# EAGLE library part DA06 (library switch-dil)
DIL/CODE SWITCH
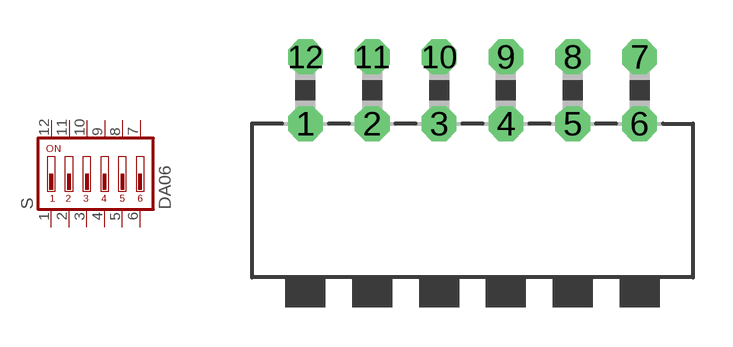
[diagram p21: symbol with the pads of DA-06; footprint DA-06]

Designator prefix S

## DA06 (MPN: MCDA06; OC_FARNELL: 9471553; OC_NEWARK: 26M1091)  [DA-06]
1  1  pas
2  2  pas
3  3  pas
4  4  pas
5  5  pas
6  6  pas
7  7  pas
8  8  pas
9  9  pas
10  10  pas
11  11  pas
12  12  pas

## Footprint DA-06 (pad centres in mm)
DIL/CODE SWITCH Mors distributor Buerklin, 17G588
drill 0.813 octagon: 1 -6.35,-1.27; 2 -3.81,-1.27; 3 -1.27,-1.27; 4 1.27,-1.27; 5 3.81,-1.27; 6 6.35,-1.27; 7 6.35,1.27; 8 3.81,1.27; 9 1.27,1.27; 10 -1.27,1.27; 11 -3.81,1.27; 12 -6.35,1.27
